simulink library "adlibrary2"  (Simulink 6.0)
settings: Solver=ode45  StartTime=0.0  StopTime=10.0  RelTol=1e-3
undefined symbols (not defined in the file or in its folder): adlibrary2, ADM, Bit, DDR, Generation, II, Location, Lower, SDRAM, SRAM, Width, XP, XPL, XRC, ZBT
libraries: xbsIndex_r3 x581, adlibrary2 x2
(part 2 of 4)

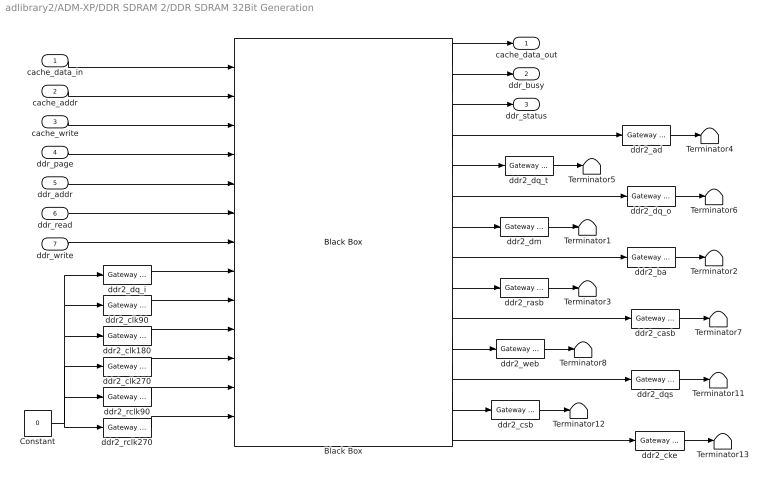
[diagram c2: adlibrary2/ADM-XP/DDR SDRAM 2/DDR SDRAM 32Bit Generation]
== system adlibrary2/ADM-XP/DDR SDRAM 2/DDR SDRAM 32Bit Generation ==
  cache_data_in : Inport  Port=1  LatchInput=off
  cache_addr : Inport  Port=2  LatchInput=off
  cache_write : Inport  Port=3  LatchInput=off
  ddr_page : Inport  Port=4  LatchInput=off
  ddr_addr : Inport  Port=5  LatchInput=off
  ddr_read : Inport  Port=6  LatchInput=off
  ddr_write : Inport  Port=7  LatchInput=off
  Black Box : xbsIndex_r3/Black Box  init_code=ddr32_config  sim_method=Inactive  show_param=on
  Constant : Constant  Value=0
  Terminator{1..8,11..13} (11 alike) : Terminator
  ddr2_ad : xbsIndex_r3/Gateway Out  hdl_port=on  timing_constraint=None  locs_specified=off  LOCs={}  needs_fixed_name=off  show_param=off
  ddr2_ba : xbsIndex_r3/Gateway Out  hdl_port=on  timing_constraint=None  locs_specified=off  LOCs={}  needs_fixed_name=off  show_param=off
  ddr2_casb : xbsIndex_r3/Gateway Out  hdl_port=on  timing_constraint=None  locs_specified=off  LOCs={}  needs_fixed_name=off  show_param=off
  ddr2_cke : xbsIndex_r3/Gateway Out  hdl_port=on  timing_constraint=None  locs_specified=off  LOCs={}  needs_fixed_name=off  show_param=off
  ddr2_clk180 : xbsIndex_r3/Gateway In  arith_type=Boolean  n_bits=64  bin_pt=0  quantization=Truncate  overflow=Wrap  period=1  timing_constraint=None  locs_specified=off  LOCs={}  needs_fixed_name=off  dbl_ovrd=off  show_param=off
  ddr2_clk270 : xbsIndex_r3/Gateway In  arith_type=Boolean  n_bits=64  bin_pt=0  quantization=Truncate  overflow=Wrap  period=1  timing_constraint=None  locs_specified=off  LOCs={}  needs_fixed_name=off  dbl_ovrd=off  show_param=off
  ddr2_clk90 : xbsIndex_r3/Gateway In  arith_type=Boolean  n_bits=64  bin_pt=0  quantization=Truncate  overflow=Wrap  period=1  timing_constraint=None  locs_specified=off  LOCs={}  needs_fixed_name=off  dbl_ovrd=off  show_param=off
  ddr2_csb : xbsIndex_r3/Gateway Out  hdl_port=on  timing_constraint=None  locs_specified=off  LOCs={}  needs_fixed_name=off  show_param=off
  ddr2_dm : xbsIndex_r3/Gateway Out  hdl_port=on  timing_constraint=None  locs_specified=off  LOCs={}  needs_fixed_name=off  show_param=off
  ddr2_dq_i : xbsIndex_r3/Gateway In  arith_type=Unsigned  n_bits=32  bin_pt=0  quantization=Truncate  overflow=Wrap  period=1  timing_constraint=None  locs_specified=off  LOCs={}  needs_fixed_name=off  dbl_ovrd=off  show_param=off
  ddr2_dq_o : xbsIndex_r3/Gateway Out  hdl_port=on  timing_constraint=None  locs_specified=off  LOCs={}  needs_fixed_name=off  show_param=off
  ddr2_dq_t : xbsIndex_r3/Gateway Out  hdl_port=on  timing_constraint=None  locs_specified=off  LOCs={}  needs_fixed_name=off  show_param=off
  ddr2_dqs : xbsIndex_r3/Gateway Out  hdl_port=on  timing_constraint=None  locs_specified=off  LOCs={}  needs_fixed_name=off  show_param=off
  ddr2_rasb : xbsIndex_r3/Gateway Out  hdl_port=on  timing_constraint=None  locs_specified=off  LOCs={}  needs_fixed_name=off  show_param=off
  ddr2_rclk270 : xbsIndex_r3/Gateway In  arith_type=Boolean  n_bits=64  bin_pt=0  quantization=Truncate  overflow=Wrap  period=1  timing_constraint=None  locs_specified=off  LOCs={}  needs_fixed_name=off  dbl_ovrd=off  show_param=off
  ddr2_rclk90 : xbsIndex_r3/Gateway In  arith_type=Boolean  n_bits=64  bin_pt=0  quantization=Truncate  overflow=Wrap  period=1  timing_constraint=None  locs_specified=off  LOCs={}  needs_fixed_name=off  dbl_ovrd=off  show_param=off
  ddr2_web : xbsIndex_r3/Gateway Out  hdl_port=on  timing_constraint=None  locs_specified=off  LOCs={}  needs_fixed_name=off  show_param=off
  cache_data_out : Outport
  ddr_busy : Outport  Port=2
  ddr_status : Outport  Port=3
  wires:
  Black Box/14 -> ddr2_cke/1
  ddr2_cke/1 -> Terminator13/1
  Black Box/13 -> ddr2_csb/1
  ddr2_csb/1 -> Terminator12/1
  ddr2_dqs/1 -> Terminator11/1
  Black Box/11 -> ddr2_web/1
  ddr2_web/1 -> Terminator8/1
  Black Box/10 -> ddr2_casb/1
  ddr2_casb/1 -> Terminator7/1
  Black Box/9 -> ddr2_rasb/1
  ddr2_rasb/1 -> Terminator3/1
  Black Box/8 -> ddr2_ba/1
  ddr2_ba/1 -> Terminator2/1
  Black Box/7 -> ddr2_dm/1
  ddr2_dm/1 -> Terminator1/1
  Black Box/6 -> ddr2_dq_o/1
  ddr2_dq_o/1 -> Terminator6/1
  Black Box/5 -> ddr2_dq_t/1
  ddr2_dq_t/1 -> Terminator5/1
  ddr2_ad/1 -> Terminator4/1
  Black Box/4 -> ddr2_ad/1
  Black Box/3 -> ddr_status/1
  Black Box/2 -> ddr_busy/1
  Black Box/1 -> cache_data_out/1
  ddr_write/1 -> Black Box/7
  ddr_read/1 -> Black Box/6
  ddr_addr/1 -> Black Box/5
  ddr_page/1 -> Black Box/4
  cache_write/1 -> Black Box/3
  cache_addr/1 -> Black Box/2
  cache_data_in/1 -> Black Box/1
  ddr2_dq_i/1 -> Black Box/8
  Constant/1 -> ddr2_dq_i/1, ddr2_clk90/1, ddr2_clk180/1, ddr2_rclk270/1, ddr2_clk270/1, ddr2_rclk90/1
  Black Box/12 -> ddr2_dqs/1
  ddr2_clk90/1 -> Black Box/9
  ddr2_clk180/1 -> Black Box/10
  ddr2_clk270/1 -> Black Box/11
  ddr2_rclk90/1 -> Black Box/12
  ddr2_rclk270/1 -> Black Box/13

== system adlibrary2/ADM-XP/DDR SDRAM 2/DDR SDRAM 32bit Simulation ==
  cache_data_in : Inport  Port=1  LatchInput=off
  cache_addr : Inport  Port=2  LatchInput=off
  cache_write : Inport  Port=3  LatchInput=off
  ddr_page : Inport  Port=4  LatchInput=off
  ddr_addr : Inport  Port=5  LatchInput=off
  ddr_read : Inport  Port=6  LatchInput=off
  ddr_write : Inport  Port=7  LatchInput=off
  Disregard Subsystem : xbsIndex_r3/Disregard Subsystem  Tag=discardX
  S-Function : S-Function  FunctionName=ddr32  Parameters=memsize
  Subsystem : adlibrary2/ADM-XRC-II/XRM DDR SDRAM /DDR SDRAM 64bit Simulation/Subsystem
  gi{0..6} (7 alike) : xbsIndex_r3/Gateway Out  hdl_port=off  timing_constraint=None  locs_specified=off  LOCs={}  needs_fixed_name=off  show_param=off
  cache_data_out : Outport
  ddr_busy : Outport  Port=2
  ddr_status : Outport  Port=3
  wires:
  cache_data_in/1 -> gi0/1
  cache_addr/1 -> gi1/1
  cache_write/1 -> gi2/1
  ddr_page/1 -> gi3/1
  ddr_addr/1 -> gi4/1
  ddr_read/1 -> gi5/1
  ddr_write/1 -> gi6/1
  gi0/1 -> S-Function/1
  gi1/1 -> S-Function/2
  gi2/1 -> S-Function/3
  gi3/1 -> S-Function/4
  gi4/1 -> S-Function/5
  gi5/1 -> S-Function/6
  gi6/1 -> S-Function/7
  S-Function/1 -> Subsystem/1
  S-Function/2 -> Subsystem/2
  S-Function/3 -> Subsystem/3
  Subsystem/1 -> cache_data_out/1
  Subsystem/2 -> ddr_busy/1
  Subsystem/3 -> ddr_status/1

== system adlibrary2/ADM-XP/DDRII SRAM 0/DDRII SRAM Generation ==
  d : Inport  Port=1  LatchInput=off
  a : Inport  Port=2  LatchInput=off
  w : Inport  Port=3  LatchInput=off
  r : Inport  Port=4  LatchInput=off
  be : Inport  Port=5  LatchInput=off
  Black Box : xbsIndex_r3/Black Box  init_code=d2sram_config  sim_method=Inactive  show_param=off
  Constant : Constant  Value=0
  Terminator{,1..3} (4 alike) : Terminator
  r0_clk180 : xbsIndex_r3/Gateway In  arith_type=Boolean  n_bits=1  bin_pt=0  quantization=Truncate  overflow=Wrap  period=1  timing_constraint=None  locs_specified=off  LOCs={}  needs_fixed_name=off  dbl_ovrd=off  show_param=off
  r0_clk270 : xbsIndex_r3/Gateway In  arith_type=Boolean  n_bits=1  bin_pt=0  quantization=Truncate  overflow=Wrap  period=1  timing_constraint=None  locs_specified=off  LOCs={}  needs_fixed_name=off  dbl_ovrd=off  show_param=off
  r0_clk90 : xbsIndex_r3/Gateway In  arith_type=Boolean  n_bits=1  bin_pt=0  quantization=Truncate  overflow=Wrap  period=1  timing_constraint=None  locs_specified=off  LOCs={}  needs_fixed_name=off  dbl_ovrd=off  show_param=off
  r0_rst : xbsIndex_r3/Gateway In  arith_type=Boolean  n_bits=1  bin_pt=0  quantization=Truncate  overflow=Wrap  period=1  timing_constraint=None  locs_specified=off  LOCs={}  needs_fixed_name=off  dbl_ovrd=off  show_param=off
  ra0 : xbsIndex_r3/Gateway Out  hdl_port=on  timing_constraint=None  locs_specified=off  LOCs={}  needs_fixed_name=off  show_param=off
  rc0 : xbsIndex_r3/Gateway Out  hdl_port=on  timing_constraint=None  locs_specified=off  LOCs={}  needs_fixed_name=off  show_param=off
  rd0_i : xbsIndex_r3/Gateway In  arith_type=Unsigned  n_bits=32  bin_pt=0  quantization=Truncate  overflow=Wrap  period=1  timing_constraint=None  locs_specified=off  LOCs={}  needs_fixed_name=off  dbl_ovrd=off  show_param=off
  rd0_o : xbsIndex_r3/Gateway Out  hdl_port=on  timing_constraint=None  locs_specified=off  LOCs={}  needs_fixed_name=off  show_param=off
  rd0_t : xbsIndex_r3/Gateway Out  hdl_port=on  timing_constraint=None  locs_specified=off  LOCs={}  needs_fixed_name=off  show_param=off
  q : Outport
  read_pending : Outport  Port=2
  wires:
  rc0/1 -> Terminator3/1
  ra0/1 -> Terminator2/1
  rd0_t/1 -> Terminator1/1
  rd0_o/1 -> Terminator/1
  Constant/1 -> rd0_i/1, r0_rst/1, r0_clk270/1, r0_clk180/1, r0_clk90/1
  be/1 -> Black Box/7
  d/1 -> Black Box/6
  a/1 -> Black Box/5
  w/1 -> Black Box/9
  r/1 -> Black Box/8
  Black Box/4 -> rd0_t/1
  Black Box/3 -> rd0_o/1
  Black Box/2 -> rc0/1
  Black Box/1 -> ra0/1
  Black Box/5 -> q/1
  r0_rst/1 -> Black Box/10
  r0_clk270/1 -> Black Box/4
  r0_clk180/1 -> Black Box/3
  r0_clk90/1 -> Black Box/2
  rd0_i/1 -> Black Box/1
  Black Box/6 -> read_pending/1

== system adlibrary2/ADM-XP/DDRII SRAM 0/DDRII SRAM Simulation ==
  d : Inport  Port=1  LatchInput=off
  a : Inport  Port=2  LatchInput=off
  w : Inport  Port=3  LatchInput=off
  r : Inport  Port=4  LatchInput=off
  be : Inport  Port=5  LatchInput=off
  Concat : xbsIndex_r3/Concat  num_inputs=2  explicit_period=off  period=1  dbl_ovrd=off
  Disregard Subsystem : xbsIndex_r3/Disregard Subsystem  Tag=discardX
  Gateway In1 : xbsIndex_r3/Gateway In  arith_type=Unsigned  n_bits=32  bin_pt=0  quantization=Truncate  overflow=Wrap  period=1  timing_constraint=None  locs_specified=off  LOCs={}  needs_fixed_name=off  dbl_ovrd=on  show_param=off
  Gateway In6 : xbsIndex_r3/Gateway In  arith_type=Boolean  n_bits=1  bin_pt=0  quantization=Truncate  overflow=Wrap  period=1  timing_constraint=None  locs_specified=off  LOCs={}  needs_fixed_name=off  dbl_ovrd=on  show_param=off
  Gateway In7 : xbsIndex_r3/Gateway In  arith_type=Unsigned  n_bits=32  bin_pt=0  quantization=Truncate  overflow=Wrap  period=1  timing_constraint=None  locs_specified=off  LOCs={}  needs_fixed_name=off  dbl_ovrd=on  show_param=off
  Gateway Out{,1..5} (6 alike) : xbsIndex_r3/Gateway Out  hdl_port=off  timing_constraint=None  locs_specified=off  LOCs={}  needs_fixed_name=off  show_param=off
  S-Function : S-Function  FunctionName=d2sram
  Slice : xbsIndex_r3/Slice  mode=Lower Bit Location + Width  nbits=32  bit1=0  base1=MSB of Input  bit0=0  base0=LSB of Input  boolean_output=off  explicit_period=off  period=1  dbl_ovrd=off
  Slice1 : xbsIndex_r3/Slice  mode=Lower Bit Location + Width  nbits=32  bit1=0  base1=MSB of Input  bit0=32  base0=LSB of Input  boolean_output=off  explicit_period=off  period=1  dbl_ovrd=off
  q : Outport
  qv : Outport  Port=2
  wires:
  Concat/1 -> q/1
  Gateway In1/1 -> Concat/2
  Gateway In7/1 -> Concat/1
  d/1 -> Slice/1, Slice1/1
  Slice/1 -> Gateway Out1/1
  Slice1/1 -> Gateway Out/1
  Gateway Out5/1 -> S-Function/6
  be/1 -> Gateway Out5/1
  S-Function/3 -> Gateway In6/1
  Gateway In6/1 -> qv/1
  S-Function/2 -> Gateway In1/1
  Gateway Out4/1 -> S-Function/5
  r/1 -> Gateway Out4/1
  Gateway Out3/1 -> S-Function/4
  Gateway Out2/1 -> S-Function/3
  Gateway Out1/1 -> S-Function/2
  Gateway Out/1 -> S-Function/1
  S-Function/1 -> Gateway In7/1
  w/1 -> Gateway Out3/1
  a/1 -> Gateway Out2/1

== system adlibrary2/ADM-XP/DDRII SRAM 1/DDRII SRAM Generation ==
  d : Inport  Port=1  LatchInput=off
  a : Inport  Port=2  LatchInput=off
  w : Inport  Port=3  LatchInput=off
  r : Inport  Port=4  LatchInput=off
  be : Inport  Port=5  LatchInput=off
  Black Box : xbsIndex_r3/Black Box  init_code=d2sram_config  sim_method=Inactive  show_param=off
  Constant : Constant  Value=0
  Terminator{,1..3} (4 alike) : Terminator
  r1_clk180 : xbsIndex_r3/Gateway In  arith_type=Boolean  n_bits=1  bin_pt=0  quantization=Truncate  overflow=Wrap  period=1  timing_constraint=None  locs_specified=off  LOCs={}  needs_fixed_name=off  dbl_ovrd=off  show_param=off
  r1_clk270 : xbsIndex_r3/Gateway In  arith_type=Boolean  n_bits=1  bin_pt=0  quantization=Truncate  overflow=Wrap  period=1  timing_constraint=None  locs_specified=off  LOCs={}  needs_fixed_name=off  dbl_ovrd=off  show_param=off
  r1_clk90 : xbsIndex_r3/Gateway In  arith_type=Boolean  n_bits=1  bin_pt=0  quantization=Truncate  overflow=Wrap  period=1  timing_constraint=None  locs_specified=off  LOCs={}  needs_fixed_name=off  dbl_ovrd=off  show_param=off
  r1_rst : xbsIndex_r3/Gateway In  arith_type=Boolean  n_bits=1  bin_pt=0  quantization=Truncate  overflow=Wrap  period=1  timing_constraint=None  locs_specified=off  LOCs={}  needs_fixed_name=off  dbl_ovrd=off  show_param=off
  ra1 : xbsIndex_r3/Gateway Out  hdl_port=on  timing_constraint=None  locs_specified=off  LOCs={}  needs_fixed_name=off  show_param=off
  rc1 : xbsIndex_r3/Gateway Out  hdl_port=on  timing_constraint=None  locs_specified=off  LOCs={}  needs_fixed_name=off  show_param=off
  rd1_i : xbsIndex_r3/Gateway In  arith_type=Unsigned  n_bits=32  bin_pt=0  quantization=Truncate  overflow=Wrap  period=1  timing_constraint=None  locs_specified=off  LOCs={}  needs_fixed_name=off  dbl_ovrd=off  show_param=off
  rd1_o : xbsIndex_r3/Gateway Out  hdl_port=on  timing_constraint=None  locs_specified=off  LOCs={}  needs_fixed_name=off  show_param=off
  rd1_t : xbsIndex_r3/Gateway Out  hdl_port=on  timing_constraint=None  locs_specified=off  LOCs={}  needs_fixed_name=off  show_param=off
  q : Outport
  read_pending : Outport  Port=2
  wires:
  Black Box/6 -> read_pending/1
  rd1_i/1 -> Black Box/1
  r1_clk90/1 -> Black Box/2
  r1_clk180/1 -> Black Box/3
  r1_clk270/1 -> Black Box/4
  r1_rst/1 -> Black Box/10
  Black Box/5 -> q/1
  Black Box/1 -> ra1/1
  Black Box/2 -> rc1/1
  Black Box/3 -> rd1_o/1
  Black Box/4 -> rd1_t/1
  r/1 -> Black Box/8
  w/1 -> Black Box/9
  a/1 -> Black Box/5
  d/1 -> Black Box/6
  be/1 -> Black Box/7
  Constant/1 -> r1_clk90/1, r1_clk180/1, r1_clk270/1, r1_rst/1, rd1_i/1
  rd1_o/1 -> Terminator/1
  rd1_t/1 -> Terminator1/1
  ra1/1 -> Terminator2/1
  rc1/1 -> Terminator3/1

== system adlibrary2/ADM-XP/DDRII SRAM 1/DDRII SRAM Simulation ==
  d : Inport  Port=1  LatchInput=off
  a : Inport  Port=2  LatchInput=off
  w : Inport  Port=3  LatchInput=off
  r : Inport  Port=4  LatchInput=off
  be : Inport  Port=5  LatchInput=off
  Concat : xbsIndex_r3/Concat  num_inputs=2  explicit_period=off  period=1  dbl_ovrd=off
  Disregard Subsystem : xbsIndex_r3/Disregard Subsystem  Tag=discardX
  Gateway In1 : xbsIndex_r3/Gateway In  arith_type=Unsigned  n_bits=32  bin_pt=0  quantization=Truncate  overflow=Wrap  period=1  timing_constraint=None  locs_specified=off  LOCs={}  needs_fixed_name=off  dbl_ovrd=on  show_param=off
  Gateway In6 : xbsIndex_r3/Gateway In  arith_type=Boolean  n_bits=1  bin_pt=0  quantization=Truncate  overflow=Wrap  period=1  timing_constraint=None  locs_specified=off  LOCs={}  needs_fixed_name=off  dbl_ovrd=on  show_param=off
  Gateway In7 : xbsIndex_r3/Gateway In  arith_type=Unsigned  n_bits=32  bin_pt=0  quantization=Truncate  overflow=Wrap  period=1  timing_constraint=None  locs_specified=off  LOCs={}  needs_fixed_name=off  dbl_ovrd=on  show_param=off
  Gateway Out{,1..5} (6 alike) : xbsIndex_r3/Gateway Out  hdl_port=off  timing_constraint=None  locs_specified=off  LOCs={}  needs_fixed_name=off  show_param=off
  S-Function : S-Function  FunctionName=d2sram
  Slice : xbsIndex_r3/Slice  mode=Lower Bit Location + Width  nbits=32  bit1=0  base1=MSB of Input  bit0=0  base0=LSB of Input  boolean_output=off  explicit_period=off  period=1  dbl_ovrd=off
  Slice1 : xbsIndex_r3/Slice  mode=Lower Bit Location + Width  nbits=32  bit1=0  base1=MSB of Input  bit0=32  base0=LSB of Input  boolean_output=off  explicit_period=off  period=1  dbl_ovrd=off
  q : Outport
  qv : Outport  Port=2
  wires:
  a/1 -> Gateway Out2/1
  w/1 -> Gateway Out3/1
  S-Function/1 -> Gateway In7/1
  Gateway Out/1 -> S-Function/1
  Gateway Out1/1 -> S-Function/2
  Gateway Out2/1 -> S-Function/3
  Gateway Out3/1 -> S-Function/4
  r/1 -> Gateway Out4/1
  Gateway Out4/1 -> S-Function/5
  S-Function/2 -> Gateway In1/1
  Gateway In6/1 -> qv/1
  S-Function/3 -> Gateway In6/1
  be/1 -> Gateway Out5/1
  Gateway Out5/1 -> S-Function/6
  Slice1/1 -> Gateway Out/1
  Slice/1 -> Gateway Out1/1
  d/1 -> Slice1/1, Slice/1
  Gateway In7/1 -> Concat/1
  Gateway In1/1 -> Concat/2
  Concat/1 -> q/1

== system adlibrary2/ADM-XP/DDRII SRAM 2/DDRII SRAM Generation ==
  d : Inport  Port=1  LatchInput=off
  a : Inport  Port=2  LatchInput=off
  w : Inport  Port=3  LatchInput=off
  r : Inport  Port=4  LatchInput=off
  be : Inport  Port=5  LatchInput=off
  Black Box : xbsIndex_r3/Black Box  init_code=d2sram_2_config  sim_method=Inactive  show_param=off
  Constant : Constant  Value=0
  Terminator{,1..3} (4 alike) : Terminator
  r2_clk180 : xbsIndex_r3/Gateway In  arith_type=Boolean  n_bits=1  bin_pt=0  quantization=Truncate  overflow=Wrap  period=1  timing_constraint=None  locs_specified=off  LOCs={}  needs_fixed_name=off  dbl_ovrd=off  show_param=off
  r2_clk270 : xbsIndex_r3/Gateway In  arith_type=Boolean  n_bits=1  bin_pt=0  quantization=Truncate  overflow=Wrap  period=1  timing_constraint=None  locs_specified=off  LOCs={}  needs_fixed_name=off  dbl_ovrd=off  show_param=off
  r2_clk90 : xbsIndex_r3/Gateway In  arith_type=Boolean  n_bits=1  bin_pt=0  quantization=Truncate  overflow=Wrap  period=1  timing_constraint=None  locs_specified=off  LOCs={}  needs_fixed_name=off  dbl_ovrd=off  show_param=off
  r2_rst : xbsIndex_r3/Gateway In  arith_type=Boolean  n_bits=1  bin_pt=0  quantization=Truncate  overflow=Wrap  period=1  timing_constraint=None  locs_specified=off  LOCs={}  needs_fixed_name=off  dbl_ovrd=off  show_param=off
  ra2 : xbsIndex_r3/Gateway Out  hdl_port=on  timing_constraint=None  locs_specified=off  LOCs={}  needs_fixed_name=off  show_param=off
  rc2 : xbsIndex_r3/Gateway Out  hdl_port=on  timing_constraint=None  locs_specified=off  LOCs={}  needs_fixed_name=off  show_param=off
  rd2_i : xbsIndex_r3/Gateway In  arith_type=Unsigned  n_bits=64  bin_pt=0  quantization=Truncate  overflow=Wrap  period=1  timing_constraint=None  locs_specified=off  LOCs={}  needs_fixed_name=off  dbl_ovrd=off  show_param=off
  rd2_o : xbsIndex_r3/Gateway Out  hdl_port=on  timing_constraint=None  locs_specified=off  LOCs={}  needs_fixed_name=off  show_param=off
  rd2_t : xbsIndex_r3/Gateway Out  hdl_port=on  timing_constraint=None  locs_specified=off  LOCs={}  needs_fixed_name=off  show_param=off
  q : Outport
  read_pending : Outport  Port=2
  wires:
  rc2/1 -> Terminator3/1
  ra2/1 -> Terminator2/1
  rd2_t/1 -> Terminator1/1
  rd2_o/1 -> Terminator/1
  Constant/1 -> rd2_i/1, r2_rst/1, r2_clk270/1, r2_clk180/1, r2_clk90/1
  be/1 -> Black Box/7
  d/1 -> Black Box/6
  a/1 -> Black Box/5
  w/1 -> Black Box/9
  r/1 -> Black Box/8
  Black Box/4 -> rd2_t/1
  Black Box/3 -> rd2_o/1
  Black Box/2 -> rc2/1
  Black Box/1 -> ra2/1
  Black Box/5 -> q/1
  r2_rst/1 -> Black Box/10
  r2_clk270/1 -> Black Box/4
  r2_clk180/1 -> Black Box/3
  r2_clk90/1 -> Black Box/2
  rd2_i/1 -> Black Box/1
  Black Box/6 -> read_pending/1

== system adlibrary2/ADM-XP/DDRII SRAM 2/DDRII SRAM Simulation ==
  d : Inport  Port=1  LatchInput=off
  a : Inport  Port=2  LatchInput=off
  w : Inport  Port=3  LatchInput=off
  r : Inport  Port=4  LatchInput=off
  be : Inport  Port=5  LatchInput=off
  Concat : xbsIndex_r3/Concat  num_inputs=2  explicit_period=off  period=1  dbl_ovrd=off
  Disregard Subsystem : xbsIndex_r3/Disregard Subsystem  Tag=discardX
  Gateway In1 : xbsIndex_r3/Gateway In  arith_type=Unsigned  n_bits=32  bin_pt=0  quantization=Truncate  overflow=Wrap  period=1  timing_constraint=None  locs_specified=off  LOCs={}  needs_fixed_name=off  dbl_ovrd=on  show_param=off
  Gateway In6 : xbsIndex_r3/Gateway In  arith_type=Boolean  n_bits=1  bin_pt=0  quantization=Truncate  overflow=Wrap  period=1  timing_constraint=None  locs_specified=off  LOCs={}  needs_fixed_name=off  dbl_ovrd=on  show_param=off
  Gateway In7 : xbsIndex_r3/Gateway In  arith_type=Unsigned  n_bits=32  bin_pt=0  quantization=Truncate  overflow=Wrap  period=1  timing_constraint=None  locs_specified=off  LOCs={}  needs_fixed_name=off  dbl_ovrd=on  show_param=off
  Gateway Out{,1..5} (6 alike) : xbsIndex_r3/Gateway Out  hdl_port=off  timing_constraint=None  locs_specified=off  LOCs={}  needs_fixed_name=off  show_param=off
  S-Function : S-Function  FunctionName=d2sram
  Slice : xbsIndex_r3/Slice  mode=Lower Bit Location + Width  nbits=32  bit1=0  base1=MSB of Input  bit0=0  base0=LSB of Input  boolean_output=off  explicit_period=off  period=1  dbl_ovrd=off
  Slice1 : xbsIndex_r3/Slice  mode=Lower Bit Location + Width  nbits=32  bit1=0  base1=MSB of Input  bit0=32  base0=LSB of Input  boolean_output=off  explicit_period=off  period=1  dbl_ovrd=off
  q : Outport
  qv : Outport  Port=2
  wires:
  Concat/1 -> q/1
  Gateway In1/1 -> Concat/2
  Gateway In7/1 -> Concat/1
  d/1 -> Slice/1, Slice1/1
  Slice/1 -> Gateway Out1/1
  Slice1/1 -> Gateway Out/1
  Gateway Out5/1 -> S-Function/6
  be/1 -> Gateway Out5/1
  S-Function/3 -> Gateway In6/1
  Gateway In6/1 -> qv/1
  S-Function/2 -> Gateway In1/1
  Gateway Out4/1 -> S-Function/5
  r/1 -> Gateway Out4/1
  Gateway Out3/1 -> S-Function/4
  Gateway Out2/1 -> S-Function/3
  Gateway Out1/1 -> S-Function/2
  Gateway Out/1 -> S-Function/1
  S-Function/1 -> Gateway In7/1
  w/1 -> Gateway Out3/1
  a/1 -> Gateway Out2/1

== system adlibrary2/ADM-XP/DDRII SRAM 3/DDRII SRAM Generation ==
  d : Inport  Port=1  LatchInput=off
  a : Inport  Port=2  LatchInput=off
  w : Inport  Port=3  LatchInput=off
  r : Inport  Port=4  LatchInput=off
  be : Inport  Port=5  LatchInput=off
  Black Box : xbsIndex_r3/Black Box  init_code=d2sram_config  sim_method=Inactive  show_param=off
  Constant : Constant  Value=0
  Terminator{,1..3} (4 alike) : Terminator
  r3_clk180 : xbsIndex_r3/Gateway In  arith_type=Boolean  n_bits=1  bin_pt=0  quantization=Truncate  overflow=Wrap  period=1  timing_constraint=None  locs_specified=off  LOCs={}  needs_fixed_name=off  dbl_ovrd=off  show_param=off
  r3_clk270 : xbsIndex_r3/Gateway In  arith_type=Boolean  n_bits=1  bin_pt=0  quantization=Truncate  overflow=Wrap  period=1  timing_constraint=None  locs_specified=off  LOCs={}  needs_fixed_name=off  dbl_ovrd=off  show_param=off
  r3_clk90 : xbsIndex_r3/Gateway In  arith_type=Boolean  n_bits=1  bin_pt=0  quantization=Truncate  overflow=Wrap  period=1  timing_constraint=None  locs_specified=off  LOCs={}  needs_fixed_name=off  dbl_ovrd=off  show_param=off
  r3_rst : xbsIndex_r3/Gateway In  arith_type=Boolean  n_bits=1  bin_pt=0  quantization=Truncate  overflow=Wrap  period=1  timing_constraint=None  locs_specified=off  LOCs={}  needs_fixed_name=off  dbl_ovrd=off  show_param=off
  ra3 : xbsIndex_r3/Gateway Out  hdl_port=on  timing_constraint=None  locs_specified=off  LOCs={}  needs_fixed_name=off  show_param=off
  rc3 : xbsIndex_r3/Gateway Out  hdl_port=on  timing_constraint=None  locs_specified=off  LOCs={}  needs_fixed_name=off  show_param=off
  rd3_i : xbsIndex_r3/Gateway In  arith_type=Unsigned  n_bits=32  bin_pt=0  quantization=Truncate  overflow=Wrap  period=1  timing_constraint=None  locs_specified=off  LOCs={}  needs_fixed_name=off  dbl_ovrd=off  show_param=off
  rd3_o : xbsIndex_r3/Gateway Out  hdl_port=on  timing_constraint=None  locs_specified=off  LOCs={}  needs_fixed_name=off  show_param=off
  rd3_t : xbsIndex_r3/Gateway Out  hdl_port=on  timing_constraint=None  locs_specified=off  LOCs={}  needs_fixed_name=off  show_param=off
  q : Outport
  read_pending : Outport  Port=2
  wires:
  rc3/1 -> Terminator3/1
  ra3/1 -> Terminator2/1
  rd3_t/1 -> Terminator1/1
  rd3_o/1 -> Terminator/1
  Constant/1 -> rd3_i/1, r3_rst/1, r3_clk270/1, r3_clk180/1, r3_clk90/1
  be/1 -> Black Box/7
  d/1 -> Black Box/6
  a/1 -> Black Box/5
  w/1 -> Black Box/9
  r/1 -> Black Box/8
  Black Box/4 -> rd3_t/1
  Black Box/3 -> rd3_o/1
  Black Box/2 -> rc3/1
  Black Box/1 -> ra3/1
  Black Box/5 -> q/1
  r3_rst/1 -> Black Box/10
  r3_clk270/1 -> Black Box/4
  r3_clk180/1 -> Black Box/3
  r3_clk90/1 -> Black Box/2
  rd3_i/1 -> Black Box/1
  Black Box/6 -> read_pending/1

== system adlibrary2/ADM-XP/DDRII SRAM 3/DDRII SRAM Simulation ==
  d : Inport  Port=1  LatchInput=off
  a : Inport  Port=2  LatchInput=off
  w : Inport  Port=3  LatchInput=off
  r : Inport  Port=4  LatchInput=off
  be : Inport  Port=5  LatchInput=off
  Concat : xbsIndex_r3/Concat  num_inputs=2  explicit_period=off  period=1  dbl_ovrd=off
  Disregard Subsystem : xbsIndex_r3/Disregard Subsystem  Tag=discardX
  Gateway In1 : xbsIndex_r3/Gateway In  arith_type=Unsigned  n_bits=32  bin_pt=0  quantization=Truncate  overflow=Wrap  period=1  timing_constraint=None  locs_specified=off  LOCs={}  needs_fixed_name=off  dbl_ovrd=on  show_param=off
  Gateway In6 : xbsIndex_r3/Gateway In  arith_type=Boolean  n_bits=1  bin_pt=0  quantization=Truncate  overflow=Wrap  period=1  timing_constraint=None  locs_specified=off  LOCs={}  needs_fixed_name=off  dbl_ovrd=on  show_param=off
  Gateway In7 : xbsIndex_r3/Gateway In  arith_type=Unsigned  n_bits=32  bin_pt=0  quantization=Truncate  overflow=Wrap  period=1  timing_constraint=None  locs_specified=off  LOCs={}  needs_fixed_name=off  dbl_ovrd=on  show_param=off
  Gateway Out{,1..5} (6 alike) : xbsIndex_r3/Gateway Out  hdl_port=off  timing_constraint=None  locs_specified=off  LOCs={}  needs_fixed_name=off  show_param=off
  S-Function : S-Function  FunctionName=d2sram
  Slice : xbsIndex_r3/Slice  mode=Lower Bit Location + Width  nbits=32  bit1=0  base1=MSB of Input  bit0=0  base0=LSB of Input  boolean_output=off  explicit_period=off  period=1  dbl_ovrd=off
  Slice1 : xbsIndex_r3/Slice  mode=Lower Bit Location + Width  nbits=32  bit1=0  base1=MSB of Input  bit0=32  base0=LSB of Input  boolean_output=off  explicit_period=off  period=1  dbl_ovrd=off
  q : Outport
  qv : Outport  Port=2
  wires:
  Concat/1 -> q/1
  Gateway In1/1 -> Concat/2
  Gateway In7/1 -> Concat/1
  d/1 -> Slice/1, Slice1/1
  Slice/1 -> Gateway Out1/1
  Slice1/1 -> Gateway Out/1
  Gateway Out5/1 -> S-Function/6
  be/1 -> Gateway Out5/1
  S-Function/3 -> Gateway In6/1
  Gateway In6/1 -> qv/1
  S-Function/2 -> Gateway In1/1
  Gateway Out4/1 -> S-Function/5
  r/1 -> Gateway Out4/1
  Gateway Out3/1 -> S-Function/4
  Gateway Out2/1 -> S-Function/3
  Gateway Out1/1 -> S-Function/2
  Gateway Out/1 -> S-Function/1
  S-Function/1 -> Gateway In7/1
  w/1 -> Gateway Out3/1
  a/1 -> Gateway Out2/1

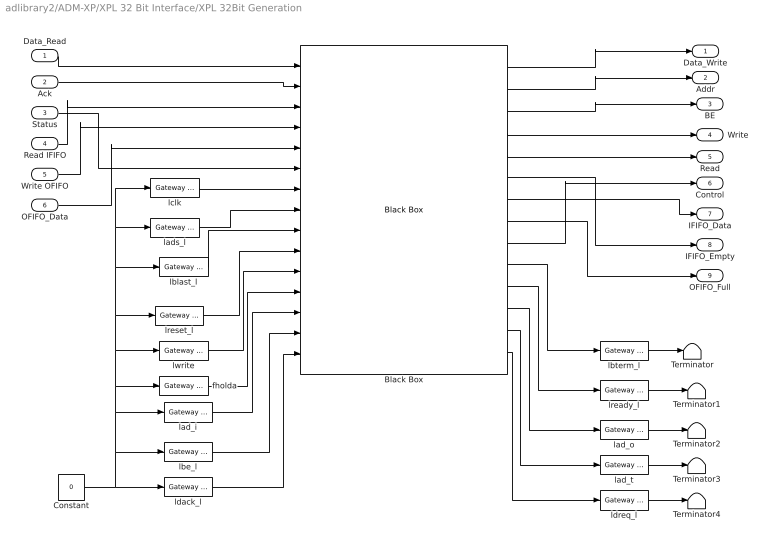
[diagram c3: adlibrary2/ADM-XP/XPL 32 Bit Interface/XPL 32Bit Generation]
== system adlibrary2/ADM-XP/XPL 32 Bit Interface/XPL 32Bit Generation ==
  Data_Read : Inport  Port=1  LatchInput=off
  Ack : Inport  Port=2  LatchInput=off
  Status : Inport  Port=3  LatchInput=off
  Read IFIFO : Inport  Port=4  LatchInput=off
  Write OFIFO : Inport  Port=5  LatchInput=off
  OFIFO_Data : Inport  Port=6  LatchInput=off
  Black Box : xbsIndex_r3/Black Box  init_code=lbif32_xpl_config  sim_method=Inactive  show_param=on
  Constant : Constant  Value=0
  Terminator{,1..4} (5 alike) : Terminator
  fholda : xbsIndex_r3/Gateway In  arith_type=Boolean  n_bits=8  bin_pt=6  quantization=Truncate  overflow=Wrap  period=1  timing_constraint=None  locs_specified=off  LOCs={}  needs_fixed_name=off  dbl_ovrd=off  show_param=off
  lad_i : xbsIndex_r3/Gateway In  arith_type=Unsigned  n_bits=64  bin_pt=0  quantization=Truncate  overflow=Wrap  period=1  timing_constraint=None  locs_specified=off  LOCs={}  needs_fixed_name=off  dbl_ovrd=off  show_param=off
  lad_o : xbsIndex_r3/Gateway Out  hdl_port=on  timing_constraint=None  locs_specified=off  LOCs={}  needs_fixed_name=off  show_param=off
  lad_t : xbsIndex_r3/Gateway Out  hdl_port=on  timing_constraint=None  locs_specified=off  LOCs={}  needs_fixed_name=off  show_param=off
  lads_l : xbsIndex_r3/Gateway In  arith_type=Boolean  n_bits=8  bin_pt=6  quantization=Truncate  overflow=Wrap  period=1  timing_constraint=None  locs_specified=off  LOCs={}  needs_fixed_name=off  dbl_ovrd=off  show_param=off
  lbe_l : xbsIndex_r3/Gateway In  arith_type=Unsigned  n_bits=8  bin_pt=0  quantization=Truncate  overflow=Wrap  period=1  timing_constraint=None  locs_specified=off  LOCs={}  needs_fixed_name=off  dbl_ovrd=off  show_param=off
  lblast_l : xbsIndex_r3/Gateway In  arith_type=Boolean  n_bits=8  bin_pt=6  quantization=Truncate  overflow=Wrap  period=1  timing_constraint=None  locs_specified=off  LOCs={}  needs_fixed_name=off  dbl_ovrd=off  show_param=off
  lbterm_l : xbsIndex_r3/Gateway Out  hdl_port=on  timing_constraint=None  locs_specified=off  LOCs={}  needs_fixed_name=off  show_param=off
  lclk : xbsIndex_r3/Gateway In  arith_type=Boolean  n_bits=8  bin_pt=6  quantization=Truncate  overflow=Wrap  period=1  timing_constraint=None  locs_specified=off  LOCs={}  needs_fixed_name=off  dbl_ovrd=off  show_param=off
  ldack_l : xbsIndex_r3/Gateway In  arith_type=Unsigned  n_bits=2  bin_pt=0  quantization=Truncate  overflow=Wrap  period=1  timing_constraint=None  locs_specified=off  LOCs={}  needs_fixed_name=off  dbl_ovrd=off  show_param=off
  ldreq_l : xbsIndex_r3/Gateway Out  hdl_port=on  timing_constraint=None  locs_specified=off  LOCs={}  needs_fixed_name=off  show_param=off
  lready_l : xbsIndex_r3/Gateway Out  hdl_port=on  timing_constraint=None  locs_specified=off  LOCs={}  needs_fixed_name=off  show_param=off
  lreset_l : xbsIndex_r3/Gateway In  arith_type=Boolean  n_bits=8  bin_pt=6  quantization=Truncate  overflow=Wrap  period=1  timing_constraint=None  locs_specified=off  LOCs={}  needs_fixed_name=off  dbl_ovrd=off  show_param=off
  lwrite : xbsIndex_r3/Gateway In  arith_type=Boolean  n_bits=8  bin_pt=6  quantization=Truncate  overflow=Wrap  period=1  timing_constraint=None  locs_specified=off  LOCs={}  needs_fixed_name=off  dbl_ovrd=off  show_param=off
  Data_Write : Outport
  Addr : Outport  Port=2
  BE : Outport  Port=3
  Write : Outport  Port=4
  Read : Outport  Port=5
  Control : Outport  Port=6
  IFIFO_Data : Outport  Port=7
  IFIFO_Empty : Outport  Port=8
  OFIFO_Full : Outport  Port=9
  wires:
  Black Box/14 -> ldreq_l/1
  Black Box/13 -> lad_t/1
  Black Box/12 -> lad_o/1
  Black Box/11 -> lready_l/1
  Black Box/10 -> lbterm_l/1
  Black Box/9 -> Control/1
  Black Box/8 -> OFIFO_Full/1
  Black Box/7 -> IFIFO_Data/1
  Black Box/6 -> IFIFO_Empty/1
  Black Box/5 -> Read/1
  Black Box/4 -> Write/1
  Black Box/3 -> BE/1
  Black Box/2 -> Addr/1
  Black Box/1 -> Data_Write/1
  lbe_l/1 -> Black Box/14
  Data_Read/1 -> Black Box/1
  Ack/1 -> Black Box/2
  Status/1 -> Black Box/6
  Read IFIFO/1 -> Black Box/3
  Write OFIFO/1 -> Black Box/4
  OFIFO_Data/1 -> Black Box/5
  lclk/1 -> Black Box/7
  lads_l/1 -> Black Box/8
  lblast_l/1 -> Black Box/9
  lreset_l/1 -> Black Box/10
  lwrite/1 -> Black Box/11
  fholda/1 -> Black Box/12
  lad_i/1 -> Black Box/13
  ldack_l/1 -> Black Box/15
  Constant/1 -> ldack_l/1, lclk/1, lads_l/1, lblast_l/1, lreset_l/1, lwrite/1, fholda/1, lad_i/1, lbe_l/1
  lbterm_l/1 -> Terminator/1
  lready_l/1 -> Terminator1/1
  lad_o/1 -> Terminator2/1
  lad_t/1 -> Terminator3/1
  ldreq_l/1 -> Terminator4/1

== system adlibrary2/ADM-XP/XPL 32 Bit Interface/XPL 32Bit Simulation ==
  Data_Read : Inport  Port=1  LatchInput=off
  Ack : Inport  Port=2  LatchInput=off
  Status : Inport  Port=3  LatchInput=off
  Read IFIFO : Inport  Port=4  LatchInput=off
  Write OFIFO : Inport  Port=5  LatchInput=off
  OFIFO_Data : Inport  Port=6  LatchInput=off
  Disregard Subsystem : xbsIndex_r3/Disregard Subsystem  Tag=discardX
  Gateway Out{,1..5} (6 alike) : xbsIndex_r3/Gateway Out  hdl_port=off  timing_constraint=None  locs_specified=off  LOCs={}  needs_fixed_name=off  show_param=off
  S-Function : S-Function  FunctionName=lbif_plx32  Parameters=program,clock_ratio
  Subsystem : Subsystem
  Data_Write : Outport
  Addr : Outport  Port=2
  BE : Outport  Port=3
  Write : Outport  Port=4
  Read : Outport  Port=5
  Control : Outport  Port=6
  IFIFO_Data : Outport  Port=7
  IFIFO_Empty : Outport  Port=8
  OFIFO_Full : Outport  Port=9
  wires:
  S-Function/9 -> Subsystem/9(In8)
  Subsystem/3(Out9) -> BE/1
  Subsystem/4(Out3) -> Write/1
  Subsystem/5(Out4) -> Read/1
  Subsystem/6(Out5) -> Control/1
  Subsystem/7(Out6) -> IFIFO_Data/1
  Subsystem/8(Out7) -> IFIFO_Empty/1
  Subsystem/9(Out8) -> OFIFO_Full/1
  Subsystem/2(Out2) -> Addr/1
  Subsystem/1(Out1) -> Data_Write/1
  S-Function/8 -> Subsystem/8(In7)
  S-Function/7 -> Subsystem/7(In6)
  S-Function/6 -> Subsystem/6(In5)
  S-Function/5 -> Subsystem/5(In4)
  S-Function/4 -> Subsystem/4(In3)
  S-Function/3 -> Subsystem/3(In9)
  S-Function/2 -> Subsystem/2(In2)
  S-Function/1 -> Subsystem/1(In1)
  Data_Read/1 -> Gateway Out/1
  Ack/1 -> Gateway Out1/1
  Status/1 -> Gateway Out2/1
  Read IFIFO/1 -> Gateway Out3/1
  Write OFIFO/1 -> Gateway Out4/1
  OFIFO_Data/1 -> Gateway Out5/1
  Gateway Out/1 -> S-Function/1
  Gateway Out1/1 -> S-Function/2
  Gateway Out2/1 -> S-Function/3
  Gateway Out3/1 -> S-Function/4
  Gateway Out4/1 -> S-Function/5
  Gateway Out5/1 -> S-Function/6

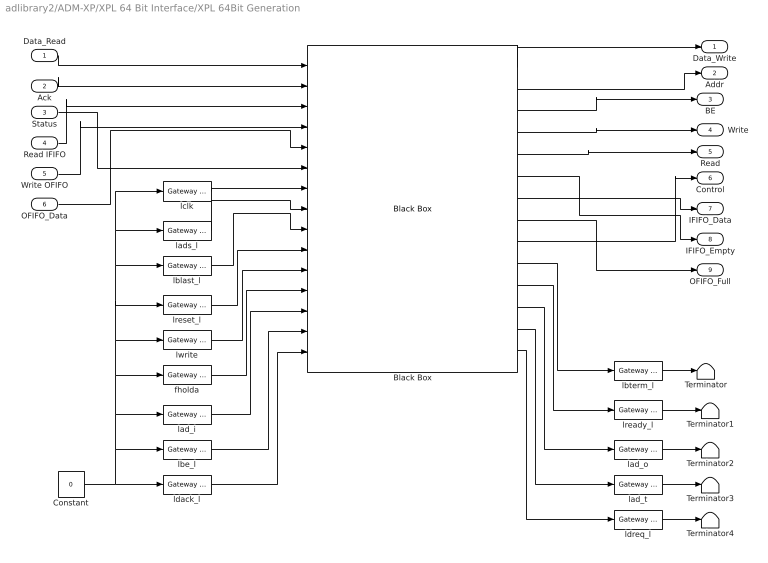
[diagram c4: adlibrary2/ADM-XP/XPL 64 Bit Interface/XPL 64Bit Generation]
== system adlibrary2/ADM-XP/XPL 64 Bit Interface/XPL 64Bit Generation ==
  Data_Read : Inport  Port=1  LatchInput=off
  Ack : Inport  Port=2  LatchInput=off
  Status : Inport  Port=3  LatchInput=off
  Read IFIFO : Inport  Port=4  LatchInput=off
  Write OFIFO : Inport  Port=5  LatchInput=off
  OFIFO_Data : Inport  Port=6  LatchInput=off
  Black Box : xbsIndex_r3/Black Box  init_code=lbif64_xpl_config  sim_method=Inactive  show_param=on
  Constant : Constant  Value=0
  Terminator{,1..4} (5 alike) : Terminator
  fholda : xbsIndex_r3/Gateway In  arith_type=Boolean  n_bits=8  bin_pt=6  quantization=Truncate  overflow=Wrap  period=1  timing_constraint=None  locs_specified=off  LOCs={}  needs_fixed_name=off  dbl_ovrd=off  show_param=off
  lad_i : xbsIndex_r3/Gateway In  arith_type=Unsigned  n_bits=64  bin_pt=0  quantization=Truncate  overflow=Wrap  period=1  timing_constraint=None  locs_specified=off  LOCs={}  needs_fixed_name=off  dbl_ovrd=off  show_param=off
  lad_o : xbsIndex_r3/Gateway Out  hdl_port=on  timing_constraint=None  locs_specified=off  LOCs={}  needs_fixed_name=off  show_param=off
  lad_t : xbsIndex_r3/Gateway Out  hdl_port=on  timing_constraint=None  locs_specified=off  LOCs={}  needs_fixed_name=off  show_param=off
  lads_l : xbsIndex_r3/Gateway In  arith_type=Boolean  n_bits=8  bin_pt=6  quantization=Truncate  overflow=Wrap  period=1  timing_constraint=None  locs_specified=off  LOCs={}  needs_fixed_name=off  dbl_ovrd=off  show_param=off
  lbe_l : xbsIndex_r3/Gateway In  arith_type=Unsigned  n_bits=8  bin_pt=0  quantization=Truncate  overflow=Wrap  period=1  timing_constraint=None  locs_specified=off  LOCs={}  needs_fixed_name=off  dbl_ovrd=off  show_param=off
  lblast_l : xbsIndex_r3/Gateway In  arith_type=Boolean  n_bits=8  bin_pt=6  quantization=Truncate  overflow=Wrap  period=1  timing_constraint=None  locs_specified=off  LOCs={}  needs_fixed_name=off  dbl_ovrd=off  show_param=off
  lbterm_l : xbsIndex_r3/Gateway Out  hdl_port=on  timing_constraint=None  locs_specified=off  LOCs={}  needs_fixed_name=off  show_param=off
  lclk : xbsIndex_r3/Gateway In  arith_type=Boolean  n_bits=8  bin_pt=6  quantization=Truncate  overflow=Wrap  period=1  timing_constraint=None  locs_specified=off  LOCs={}  needs_fixed_name=off  dbl_ovrd=off  show_param=off
  ldack_l : xbsIndex_r3/Gateway In  arith_type=Unsigned  n_bits=2  bin_pt=0  quantization=Truncate  overflow=Wrap  period=1  timing_constraint=None  locs_specified=off  LOCs={}  needs_fixed_name=off  dbl_ovrd=off  show_param=off
  ldreq_l : xbsIndex_r3/Gateway Out  hdl_port=on  timing_constraint=None  locs_specified=off  LOCs={}  needs_fixed_name=off  show_param=off
  lready_l : xbsIndex_r3/Gateway Out  hdl_port=on  timing_constraint=None  locs_specified=off  LOCs={}  needs_fixed_name=off  show_param=off
  lreset_l : xbsIndex_r3/Gateway In  arith_type=Boolean  n_bits=8  bin_pt=6  quantization=Truncate  overflow=Wrap  period=1  timing_constraint=None  locs_specified=off  LOCs={}  needs_fixed_name=off  dbl_ovrd=off  show_param=off
  lwrite : xbsIndex_r3/Gateway In  arith_type=Boolean  n_bits=8  bin_pt=6  quantization=Truncate  overflow=Wrap  period=1  timing_constraint=None  locs_specified=off  LOCs={}  needs_fixed_name=off  dbl_ovrd=off  show_param=off
  Data_Write : Outport
  Addr : Outport  Port=2
  BE : Outport  Port=3
  Write : Outport  Port=4
  Read : Outport  Port=5
  Control : Outport  Port=6
  IFIFO_Data : Outport  Port=7
  IFIFO_Empty : Outport  Port=8
  OFIFO_Full : Outport  Port=9
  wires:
  Black Box/13 -> lad_t/1
  Black Box/12 -> lad_o/1
  Black Box/11 -> lready_l/1
  Black Box/10 -> lbterm_l/1
  Black Box/9 -> Control/1
  Black Box/8 -> OFIFO_Full/1
  Black Box/7 -> IFIFO_Data/1
  Black Box/6 -> IFIFO_Empty/1
  Black Box/5 -> Read/1
  Black Box/4 -> Write/1
  Black Box/3 -> BE/1
  Black Box/14 -> ldreq_l/1
  ldreq_l/1 -> Terminator4/1
  lad_t/1 -> Terminator3/1
  lad_o/1 -> Terminator2/1
  lready_l/1 -> Terminator1/1
  lbterm_l/1 -> Terminator/1
  Constant/1 -> lbe_l/1, lad_i/1, fholda/1, lwrite/1, lreset_l/1, lblast_l/1, lads_l/1, lclk/1, ldack_l/1
  ldack_l/1 -> Black Box/15
  lad_i/1 -> Black Box/13
  fholda/1 -> Black Box/12
  lwrite/1 -> Black Box/11
  lreset_l/1 -> Black Box/10
  lblast_l/1 -> Black Box/9
  lads_l/1 -> Black Box/8
  lclk/1 -> Black Box/7
  Black Box/2 -> Addr/1
  Black Box/1 -> Data_Write/1
  OFIFO_Data/1 -> Black Box/5
  Write OFIFO/1 -> Black Box/4
  Read IFIFO/1 -> Black Box/3
  Status/1 -> Black Box/6
  Ack/1 -> Black Box/2
  Data_Read/1 -> Black Box/1
  lbe_l/1 -> Black Box/14

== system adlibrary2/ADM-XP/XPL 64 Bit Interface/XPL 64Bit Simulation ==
  Data_Read : Inport  Port=1  LatchInput=off
  Ack : Inport  Port=2  LatchInput=off
  Status : Inport  Port=3  LatchInput=off
  Read IFIFO : Inport  Port=4  LatchInput=off
  Write OFIFO : Inport  Port=5  LatchInput=off
  OFIFO_Data : Inport  Port=6  LatchInput=off
  Disregard Subsystem : xbsIndex_r3/Disregard Subsystem  Tag=discardX
  Gateway Out{,1..8} (9 alike) : xbsIndex_r3/Gateway Out  hdl_port=off  timing_constraint=None  locs_specified=off  LOCs={}  needs_fixed_name=off  show_param=off
  S-Function : S-Function  FunctionName=lbif_xpl64  Parameters=program,clock_ratio
  Slice : xbsIndex_r3/Slice  mode=Lower Bit Location + Width  nbits=32  bit1=0  base1=MSB of Input  bit0=0  base0=LSB of Input  boolean_output=off  explicit_period=off  period=1  dbl_ovrd=off
  Slice1 : xbsIndex_r3/Slice  mode=Lower Bit Location + Width  nbits=32  bit1=0  base1=MSB of Input  bit0=32  base0=LSB of Input  boolean_output=off  explicit_period=off  period=1  dbl_ovrd=off
  Slice2 : xbsIndex_r3/Slice  mode=Lower Bit Location + Width  nbits=32  bit1=0  base1=MSB of Input  bit0=0  base0=LSB of Input  boolean_output=off  explicit_period=off  period=1  dbl_ovrd=off
  Slice3 : xbsIndex_r3/Slice  mode=Lower Bit Location + Width  nbits=32  bit1=0  base1=MSB of Input  bit0=32  base0=LSB of Input  boolean_output=off  explicit_period=off  period=1  dbl_ovrd=off
  Slice4 : xbsIndex_r3/Slice  mode=Lower Bit Location + Width  nbits=32  bit1=0  base1=MSB of Input  bit0=0  base0=LSB of Input  boolean_output=off  explicit_period=off  period=1  dbl_ovrd=off
  Slice5 : xbsIndex_r3/Slice  mode=Lower Bit Location + Width  nbits=32  bit1=0  base1=MSB of Input  bit0=32  base0=LSB of Input  boolean_output=off  explicit_period=off  period=1  dbl_ovrd=off
  Subsystem : Subsystem
  Data_Write : Outport
  Addr : Outport  Port=2
  BE : Outport  Port=3
  Write : Outport  Port=4
  Read : Outport  Port=5
  Control : Outport  Port=6
  IFIFO_Data : Outport  Port=7
  IFIFO_Empty : Outport  Port=8
  OFIFO_Full : Outport  Port=9
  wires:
  Subsystem/1(Out1) -> Data_Write/1
  Subsystem/2(Out2) -> Addr/1
  Subsystem/3(Out3) -> BE/1
  Subsystem/4(Out4) -> Write/1
  Subsystem/5(Out5) -> Read/1
  Subsystem/6(Out6) -> Control/1
  Subsystem/7(Out7) -> IFIFO_Data/1
  Subsystem/8(Out8) -> IFIFO_Empty/1
  Subsystem/9(Out9) -> OFIFO_Full/1
  S-Function/10 -> Subsystem/10(ififo_data1)
  S-Function/11 -> Subsystem/11(ififo_empty)
  S-Function/12 -> Subsystem/12(ofifo_full)
  S-Function/9 -> Subsystem/9(ififo_data0)
  S-Function/8 -> Subsystem/8(control1)
  S-Function/7 -> Subsystem/7(control0)
  S-Function/6 -> Subsystem/6(read)
  S-Function/5 -> Subsystem/5(write)
  S-Function/4 -> Subsystem/4(be)
  S-Function/3 -> Subsystem/3(addr)
  S-Function/2 -> Subsystem/2(data_write1)
  S-Function/1 -> Subsystem/1(data_write0)
  Gateway Out8/1 -> S-Function/9
  Gateway Out5/1 -> S-Function/8
  Slice5/1 -> Gateway Out8/1
  Slice4/1 -> Gateway Out5/1
  Gateway Out4/1 -> S-Function/7
  Gateway Out3/1 -> S-Function/6
  Gateway Out7/1 -> S-Function/5
  Gateway Out2/1 -> S-Function/4
  Slice3/1 -> Gateway Out7/1
  Slice2/1 -> Gateway Out2/1
  Gateway Out1/1 -> S-Function/3
  Gateway Out6/1 -> S-Function/2
  Gateway Out/1 -> S-Function/1
  Slice1/1 -> Gateway Out6/1
  Slice/1 -> Gateway Out/1
  OFIFO_Data/1 -> Slice5/1, Slice4/1
  Write OFIFO/1 -> Gateway Out4/1
  Read IFIFO/1 -> Gateway Out3/1
  Status/1 -> Slice3/1, Slice2/1
  Ack/1 -> Gateway Out1/1
  Data_Read/1 -> Slice1/1, Slice/1

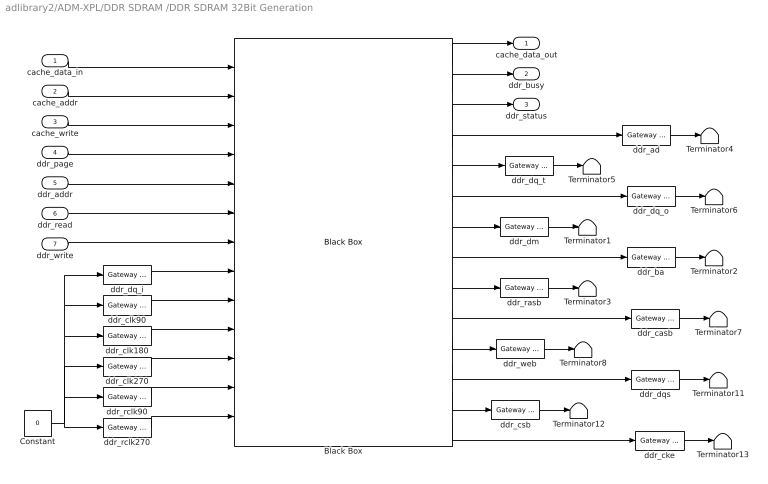
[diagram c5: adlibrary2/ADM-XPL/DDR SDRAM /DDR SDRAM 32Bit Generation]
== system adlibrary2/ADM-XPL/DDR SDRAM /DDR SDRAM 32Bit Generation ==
  cache_data_in : Inport  Port=1  LatchInput=off
  cache_addr : Inport  Port=2  LatchInput=off
  cache_write : Inport  Port=3  LatchInput=off
  ddr_page : Inport  Port=4  LatchInput=off
  ddr_addr : Inport  Port=5  LatchInput=off
  ddr_read : Inport  Port=6  LatchInput=off
  ddr_write : Inport  Port=7  LatchInput=off
  Black Box : xbsIndex_r3/Black Box  init_code=ddr32_config  sim_method=Inactive  show_param=on
  Constant : Constant  Value=0
  Terminator{1..8,11..13} (11 alike) : Terminator
  ddr_ad : xbsIndex_r3/Gateway Out  hdl_port=on  timing_constraint=None  locs_specified=off  LOCs={}  needs_fixed_name=off  show_param=off
  ddr_ba : xbsIndex_r3/Gateway Out  hdl_port=on  timing_constraint=None  locs_specified=off  LOCs={}  needs_fixed_name=off  show_param=off
  ddr_casb : xbsIndex_r3/Gateway Out  hdl_port=on  timing_constraint=None  locs_specified=off  LOCs={}  needs_fixed_name=off  show_param=off
  ddr_cke : xbsIndex_r3/Gateway Out  hdl_port=on  timing_constraint=None  locs_specified=off  LOCs={}  needs_fixed_name=off  show_param=off
  ddr_clk180 : xbsIndex_r3/Gateway In  arith_type=Boolean  n_bits=64  bin_pt=0  quantization=Truncate  overflow=Wrap  period=1  timing_constraint=None  locs_specified=off  LOCs={}  needs_fixed_name=off  dbl_ovrd=off  show_param=off
  ddr_clk270 : xbsIndex_r3/Gateway In  arith_type=Boolean  n_bits=64  bin_pt=0  quantization=Truncate  overflow=Wrap  period=1  timing_constraint=None  locs_specified=off  LOCs={}  needs_fixed_name=off  dbl_ovrd=off  show_param=off
  ddr_clk90 : xbsIndex_r3/Gateway In  arith_type=Boolean  n_bits=64  bin_pt=0  quantization=Truncate  overflow=Wrap  period=1  timing_constraint=None  locs_specified=off  LOCs={}  needs_fixed_name=off  dbl_ovrd=off  show_param=off
  ddr_csb : xbsIndex_r3/Gateway Out  hdl_port=on  timing_constraint=None  locs_specified=off  LOCs={}  needs_fixed_name=off  show_param=off
  ddr_dm : xbsIndex_r3/Gateway Out  hdl_port=on  timing_constraint=None  locs_specified=off  LOCs={}  needs_fixed_name=off  show_param=off
  ddr_dq_i : xbsIndex_r3/Gateway In  arith_type=Unsigned  n_bits=32  bin_pt=0  quantization=Truncate  overflow=Wrap  period=1  timing_constraint=None  locs_specified=off  LOCs={}  needs_fixed_name=off  dbl_ovrd=off  show_param=off
  ddr_dq_o : xbsIndex_r3/Gateway Out  hdl_port=on  timing_constraint=None  locs_specified=off  LOCs={}  needs_fixed_name=off  show_param=off
  ddr_dq_t : xbsIndex_r3/Gateway Out  hdl_port=on  timing_constraint=None  locs_specified=off  LOCs={}  needs_fixed_name=off  show_param=off
  ddr_dqs : xbsIndex_r3/Gateway Out  hdl_port=on  timing_constraint=None  locs_specified=off  LOCs={}  needs_fixed_name=off  show_param=off
  ddr_rasb : xbsIndex_r3/Gateway Out  hdl_port=on  timing_constraint=None  locs_specified=off  LOCs={}  needs_fixed_name=off  show_param=off
  ddr_rclk270 : xbsIndex_r3/Gateway In  arith_type=Boolean  n_bits=64  bin_pt=0  quantization=Truncate  overflow=Wrap  period=1  timing_constraint=None  locs_specified=off  LOCs={}  needs_fixed_name=off  dbl_ovrd=off  show_param=off
  ddr_rclk90 : xbsIndex_r3/Gateway In  arith_type=Boolean  n_bits=64  bin_pt=0  quantization=Truncate  overflow=Wrap  period=1  timing_constraint=None  locs_specified=off  LOCs={}  needs_fixed_name=off  dbl_ovrd=off  show_param=off
  ddr_web : xbsIndex_r3/Gateway Out  hdl_port=on  timing_constraint=None  locs_specified=off  LOCs={}  needs_fixed_name=off  show_param=off
  cache_data_out : Outport
  ddr_busy : Outport  Port=2
  ddr_status : Outport  Port=3
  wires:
  Black Box/14 -> ddr_cke/1
  ddr_cke/1 -> Terminator13/1
  Black Box/13 -> ddr_csb/1
  ddr_csb/1 -> Terminator12/1
  ddr_dqs/1 -> Terminator11/1
  Black Box/11 -> ddr_web/1
  ddr_web/1 -> Terminator8/1
  Black Box/10 -> ddr_casb/1
  ddr_casb/1 -> Terminator7/1
  Black Box/9 -> ddr_rasb/1
  ddr_rasb/1 -> Terminator3/1
  Black Box/8 -> ddr_ba/1
  ddr_ba/1 -> Terminator2/1
  Black Box/7 -> ddr_dm/1
  ddr_dm/1 -> Terminator1/1
  Black Box/6 -> ddr_dq_o/1
  ddr_dq_o/1 -> Terminator6/1
  Black Box/5 -> ddr_dq_t/1
  ddr_dq_t/1 -> Terminator5/1
  ddr_ad/1 -> Terminator4/1
  Black Box/4 -> ddr_ad/1
  Black Box/3 -> ddr_status/1
  Black Box/2 -> ddr_busy/1
  Black Box/1 -> cache_data_out/1
  ddr_write/1 -> Black Box/7
  ddr_read/1 -> Black Box/6
  ddr_addr/1 -> Black Box/5
  ddr_page/1 -> Black Box/4
  cache_write/1 -> Black Box/3
  cache_addr/1 -> Black Box/2
  cache_data_in/1 -> Black Box/1
  ddr_dq_i/1 -> Black Box/8
  Constant/1 -> ddr_dq_i/1, ddr_clk90/1, ddr_clk180/1, ddr_rclk270/1, ddr_clk270/1, ddr_rclk90/1
  Black Box/12 -> ddr_dqs/1
  ddr_clk90/1 -> Black Box/9
  ddr_clk180/1 -> Black Box/10
  ddr_clk270/1 -> Black Box/11
  ddr_rclk90/1 -> Black Box/12
  ddr_rclk270/1 -> Black Box/13

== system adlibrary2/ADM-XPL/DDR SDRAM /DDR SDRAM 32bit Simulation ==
  cache_data_in : Inport  Port=1  LatchInput=off
  cache_addr : Inport  Port=2  LatchInput=off
  cache_write : Inport  Port=3  LatchInput=off
  ddr_page : Inport  Port=4  LatchInput=off
  ddr_addr : Inport  Port=5  LatchInput=off
  ddr_read : Inport  Port=6  LatchInput=off
  ddr_write : Inport  Port=7  LatchInput=off
  Disregard Subsystem : xbsIndex_r3/Disregard Subsystem  Tag=discardX
  S-Function : S-Function  FunctionName=ddr32  Parameters=memsize
  Subsystem : Subsystem
  gi{0..6} (7 alike) : xbsIndex_r3/Gateway Out  hdl_port=off  timing_constraint=None  locs_specified=off  LOCs={}  needs_fixed_name=off  show_param=off
  cache_data_out : Outport
  ddr_busy : Outport  Port=2
  ddr_status : Outport  Port=3
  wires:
  gi6/1 -> S-Function/7
  gi5/1 -> S-Function/6
  gi4/1 -> S-Function/5
  gi3/1 -> S-Function/4
  gi2/1 -> S-Function/3
  gi1/1 -> S-Function/2
  gi0/1 -> S-Function/1
  ddr_write/1 -> gi6/1
  ddr_read/1 -> gi5/1
  ddr_addr/1 -> gi4/1
  ddr_page/1 -> gi3/1
  cache_write/1 -> gi2/1
  cache_addr/1 -> gi1/1
  cache_data_in/1 -> gi0/1
  S-Function/1 -> Subsystem/1(In1)
  S-Function/2 -> Subsystem/2(In2)
  S-Function/3 -> Subsystem/3(In3)
  Subsystem/1(Out1) -> cache_data_out/1
  Subsystem/2(Out2) -> ddr_busy/1
  Subsystem/3(Out3) -> ddr_status/1
